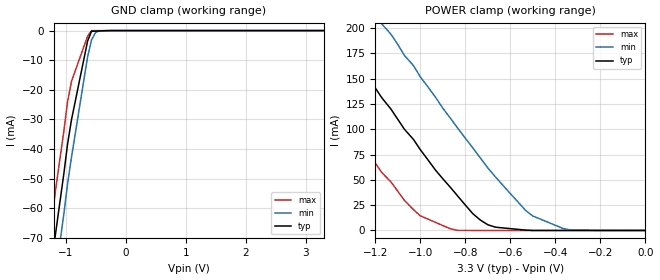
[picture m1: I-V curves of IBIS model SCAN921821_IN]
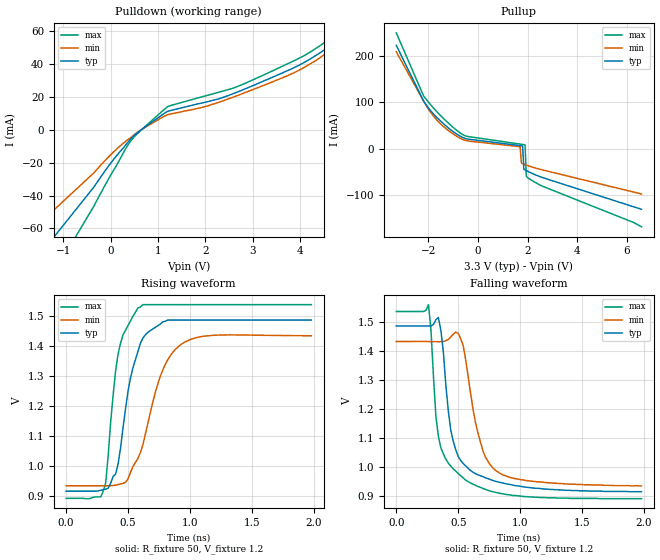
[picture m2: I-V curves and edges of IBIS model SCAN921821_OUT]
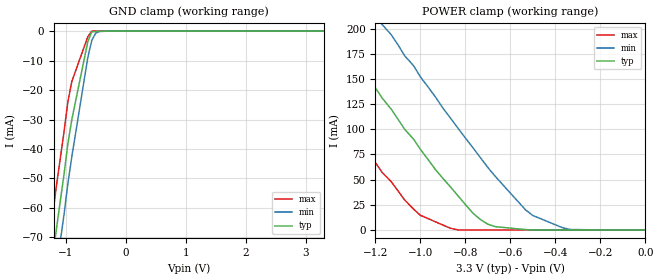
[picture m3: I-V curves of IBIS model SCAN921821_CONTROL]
|   National Semiconductor Corporation
|   IBIS Model of SCAN921821TSM
|   Dual 18-Bit BUS LVDS Serializer with Pre-emphasis,
|   IEEE 1149.1 (JTAG), and At-Speed BIST - 15-66 MHz
|   100 Ball FBGA Package
[IBIS Ver]   3.2
[Comment Char]   |_char
[File name]   scan921821tsm.ibs
[File Rev]   1.0
[Date]   04/06/04
[Source]
SPICE to IBIS Translation
[Notes]
Rev1.0 - Initial draft;
-The model cover zero pre-emphasis case only;
Created by dglisic;
[Disclaimer]
(C) Copyright National Semiconductor Corporation 2002
   All rights reserved
   National Semiconductor Corporation hereby grants
the user of this IBIS model a non-exclusive, nontransferable
license to use this IBIS model under the following terms.
Before using this IBIS model, the user should read this
license.  If the user does not accept these terms,  the
IBIS model should be returned to National within 30 days.
   The user is granted this license only to use the
IBIS model and is not granted rights to sell, load, rent,
lease or license the IBIS model in whole or in part, or in
modified form to anyone other than user. User may modify
the IBIS model to suit its specific applications but rights
to derivative works and such modifications shall belong to
National.
   This IBIS model is provided on an "AS IS" basis and
National makes absolutely no warranty with respect to the
information contained herein.NATIONAL DISCLAIMS AND CUSTOMER
WAIVES ALL WARRANTIES, EXPRESS OR IMPLIED, INCLUDING
WARRANTIES OF MERCHANTABILITY OR FITNESS FOR A PARTICULAR
PURPOSE. The entire risk as to quality and performance is
with the Customer. ACCORDINGLY, IN NO EVENT SHALL THE
COMPANY BE LIABLE FOR ANY DAMAGES, WHETHER IN CONTRACT OR
TORT,INCLUDING ANY LOST PROFITS OR OTHER INCIDENTAL,
CONSEQUENTIAL, EXEMPLARY, OR PUNITIVE DAMAGES ARISING OUT
OF THE USE OR APPLICATION OF THE IBIS model provided in
this package.Further, National reserves the right to make
changes without notice to any product herein to improve
reliability, function, or design. National does not convey
any license under patent rights or any other intellectual
property rights, including those of third parties.
   National is not obligated to provide maintenance or support
for the licensed IBIS model.
Contact National at ATTN:INTERFACE APPLICATIONS/IBIS MODELS.
5 Foden Road, M/S 03-03, South Porltand, ME 04106
(207) 541-6031
[Copyright]
(c) Copyright 2002 National Semiconductor Corp.
[Component]   SCAN921821TSM
Si_location Pin
Timing_location Pin
[Manufacturer]   National Semiconductor Corp.
[Package]
|   TYP   MIN   MAX
R_pkg   0.451   0.428   0.605
L_pkg   3.235nH   2.783n   4.687n
C_pkg   0.090pF   0.075p   0.158p
[Pin]   signal_name   model_name   R_pin   L_pin   C_pin
A1   BISTB   SCAN921821_CONTROL   0.451   3.235n  0.090p
A2   PVSS   GND   0.451   3.235n  0.090p
A3   DOUTBN  SCAN921821_OUT   0.494   3.212n  0.082p
A4   AVDD   POWER   0.469   3.235n  0.090p
A5   ENB   SCAN921821_CONTROL   0.431   2.989n  0.087p
A6   AVDD   POWER   0.429   3.125n  0.087p
A7   DOUTAN  SCAN921821_OUT   0.429   3.199n  0.087p
A8   DOUTAP  SCAN921821_OUT   0.445   3.581n  0.089p
A9   AVDD   POWER   0.463   3.856n  0.108p
A10   ENA   SCAN921821_CONTROL   0.451   3.235n  0.090p
B1   DINB16  SCAN921821_IN   0.451   3.235n  0.090p
B2   SYNCB   SCAN921821_CONTROL   0.451   3.235n  0.090p
B3   AVDD   POWER   0.588   3.928n  0.158p
B4   DOUTBP  SCAN921821_OUT   0.485   2.948n  0.082p
B5   AVDD   POWER   0.456   3.235n  0.090p
B6   PEMB1   SCAN921821_CONTROL   0.454   3.235n  0.090p
B7   AVSS   GND   0.428   3.235n  0.090p
B8   PEMB0   SCAN921821_CONTROL   0.477   3.235n  0.090p
B9   PEMA1   SCAN921821_CONTROL   0.451   3.235n  0.090p
B10   BISTA   SCAN921821_CONTROL   0.451   3.235n  0.090p
C1   DINB14  SCAN921821_IN   0.451   3.235n  0.090p
C2   DVDD   POWER   0.451   3.235n  0.090p
C3   DVSS   GND   0.451   3.235n  0.090p
C4   AVSS   GND   0.605   3.235n  0.090p
C5   AVSS   GND   0.544   3.235n  0.090p
C6   AVSS   GND   0.464   3.235n  0.090p
C7   AVDD   POWER   0.447   3.235n  0.090p
C8   PEMA2   SCAN921821_CONTROL   0.451   3.235n  0.090p
C9   SYNCA   SCAN921821_CONTROL   0.451   3.235n  0.090p
C10   DINA16  SCAN921821_IN   0.451   3.235n  0.090p
D1   DINB13  SCAN921821_IN   0.556   3.235n  0.090p
D2   DINB12  SCAN921821_IN   0.451   3.235n  0.090p
D3   DINB17  SCAN921821_IN   0.451   3.235n  0.090p
D4   DVDD   POWER   0.451   3.235n  0.090p
D5   PVDD   POWER   0.451   3.235n  0.090p
D6   PEMA0   SCAN921821_CONTROL   0.451   3.235n  0.090p
D7   AVSS   GND   0.451   3.235n  0.090p
D8   DINA17  SCAN921821_IN   0.451   3.235n  0.090p
D9   DINA15  SCAN921821_IN   0.451   3.235n  0.090p
D10   DINA13  SCAN921821_IN   0.451   3.235n  0.090p
E1   DINB11  SCAN921821_IN   0.451   3.235n  0.090p
E2   DINB9   SCAN921821_IN   0.451   3.235n  0.090p
E3   DINB15  SCAN921821_IN   0.451   3.235n  0.090p
E4   DVSS   GND   0.451   3.235n  0.090p
E5   DINB8   SCAN921821_IN   0.451   3.235n  0.090p
E6   PEMB2   SCAN921821_CONTROL   0.600   3.235n  0.090p
E7   DVSS   GND   0.451   3.235n  0.090p
E8   DINA14  SCAN921821_IN   0.451   3.235n  0.090p
E9   DINA12  SCAN921821_IN   0.451   3.235n  0.090p
E10   DINA9   SCAN921821_IN   0.451   3.235n  0.090p
F1   DINB10  SCAN921821_IN   0.451   3.235n  0.090p
F2   DINB7   SCAN921821_IN   0.451   3.235n  0.090p
F3   DINB5   SCAN921821_IN   0.451   3.235n  0.090p
F4   DVSS   GND   0.451   3.235n  0.090p
F5   PVDD   POWER   0.451   3.235n  0.090p
F6   DINA11  SCAN921821_IN   0.451   3.235n  0.090p
F7   DVSS   GND   0.451   3.235n  0.090p
F8   DINA4   SCAN921821_IN   0.451   3.235n  0.090p
F9   DINA10  SCAN921821_IN   0.451   3.235n  0.090p
F10   DINA8   SCAN921821_IN   0.451   3.235n  0.090p
G1   DINB6   SCAN921821_IN   0.451   3.235n  0.090p
G2   DINB4   SCAN921821_IN   0.451   3.235n  0.090p
G3   DINB2   SCAN921821_IN   0.451   3.235n  0.090p
G4   DVSS   GND   0.451   3.235n  0.090p
G5   DVDD   POWER   0.451   3.235n  0.090p
G6   DVDD   POWER   0.451   3.235n  0.090p
G7   DINA1   SCAN921821_IN   0.451   3.235n  0.090p
G8   DINA2   SCAN921821_IN   0.451   3.235n  0.090p
G9   DINA7   SCAN921821_IN   0.451   3.235n  0.090p
G10   DINA6   SCAN921821_IN   0.451   3.235n  0.090p
H1   DINB3   SCAN921821_IN   0.451   3.235n  0.090p
H2   DINB1   SCAN921821_IN   0.451   3.235n  0.090p
H3   TxCLK   SCAN921821_IN   0.451   3.235n  0.090p
H4   DVSS   GND   0.451   3.235n  0.090p
H5   TCK   SCAN921821_CONTROL   0.451   3.235n  0.090p
H6   PVDD   POWER   0.451   3.235n  0.090p
H7   PVSS   GND   0.451   3.235n  0.090p
H8   DVSS   GND   0.451   3.235n  0.090p
H9   DINA0   SCAN921821_IN   0.451   3.235n  0.090p
H10   DINA5   SCAN921821_IN   0.451   3.235n  0.090p
J1   DINB0   SCAN921821_IN   0.451   3.235n  0.090p
J2   PWDNA*  SCAN921821_CONTROL   0.451   3.235n  0.090p
J3   DVDD   POWER   0.451   3.235n  0.090p
J4   TRST*   SCAN921821_CONTROL   0.451   3.235n  0.090p
J5   PVDD   POWER   0.451   3.235n  0.090p
J6   PVSS   GND   0.451   3.235n  0.090p
J7   PVDD   POWER   0.451   3.235n  0.090p
J8   NC   NC   0.451   3.235n  0.090p
J9   DVDD   POWER   0.451   3.235n  0.090p
J10   DINA3   SCAN921821_IN   0.451   3.235n  0.090p
K1   DVSS   GND   0.451   3.235n  0.090p
K2   TDI   SCAN921821_CONTROL   0.451   3.235n  0.090p
K3   TMS   SCAN921821_CONTROL   0.451   3.235n  0.090p
K4   DVSS   GND   0.451   3.235n  0.090p
K5   TDO   NC   0.451   3.235n  0.090p
K6   DVDD   POWER   0.451   3.235n  0.090p
K7   PVSS   GND   0.451   3.235n  0.090p
K8   PVSS   GND   0.451   3.235n  0.090p
K9   PWDNB*  SCAN921821_CONTROL   0.451   3.235n  0.090p
K10   DVDD   POWER   0.451   3.235n  0.090p
[Diff Pin] inv_pin   vdiff   tdelay_typ   tdelay_min   tdelay_max
| The '+' pin is Diff_pin and the '-' pin is the inv_pin
| Receiver Vth = +/-100mV
A8   A7   NA   0   0   0
B4   A3   NA   0   0   0
| Models and submodels in the file (3): SCAN921821_IN (Input), SCAN921821_OUT (Output), SCAN921821_CONTROL (Input)
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[Model]   SCAN921821_IN
Model_type Input
Vinh=2.0
Vinl=0.8
C_comp   4.0pF   4.0pF   4.0pF
[Temperature Range] 25   85   -40
[Voltage Range]   3.3   3.15   3.45
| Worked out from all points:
|   GND clamp passes 1 mA (typ) near -0.58 V on its own axis
|   POWER clamp passes 1 mA (typ) near -0.56 V on its own axis
[GND Clamp]
|V(groundclamp)   I(typ)   I(min)   I(max)
-3.3V     -416mA     -429mA     -402mA
-1.3V     -89.7mA    -104mA     -74.9mA
-1.23V    -79.3mA    -93mA      -64.5mA
-1.17V    -69.1mA    -82.7mA    -54.4mA
-1.1V     -58.8mA    -72.5mA    -44.3mA
-1.03V    -48.6mA    -62.2mA    -34.2mA
-967mV    -38.4mA    -51.9mA    -24.1mA
-900mV    -30mA      -42.6mA    -17.1mA
-633mV    -3.57mA    -8.92mA    -1.9mA
-567mV    -239uA     -3.14mA    -420nA
-433mV    -133uA     -61.9uA    -233nA
3.3V      21.4pA     6.6nA      19.4pA
[POWER Clamp]
|Vtable   I(typ)   I(min)   I(max)
-3.3V     826mA      900mA      750mA
-1.63V    280mA      354mA      203mA
-1.6V     269mA      344mA      193mA
-1.37V    194mA      268mA      118mA
-1.17V    131mA      204mA      57.1mA
-1.13V    120mA      194mA      48mA
-1V       80mA       152mA      14.5mA
-833mV    33.9mA     101mA      60uA
-700mV    5.68mA     61.9mA     6.68uA
-533mV    372uA      20mA       1.71nA
-366mV    1.1uA      2.03mA     12.8pA
0V        6.66pA     6.59nA     6.3pA
[Model]   SCAN921821_OUT
Model_type Output
Vref=1.2
Vmeas=1.2
Rref=50   | 100 Ohms Across Outputs OUTP and OUTM
Cref=0p
C_comp   3.122pF   3.122pF   3.122pF
[Temperature Range] 25   85   -40
[Voltage Range]   3.3   3.15   3.45
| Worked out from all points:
|   slope of the pulldown table from 0 to 0.495 V, typ, clamps not added: 29.3 ohm
|   slope of the pullup table from 0 to 0.495 V, typ, clamps not added: 151 ohm
|   falling waveform, R_fixture 50, V_fixture 1.2: 20-80 % time 126ps typ, 147ps min, 123ps max; typ from 1.49 V to 0.916 V
|   rising waveform, R_fixture 50, V_fixture 1.2: 20-80 % time 144ps typ, 207ps min, 102ps max; typ from 0.917 V to 1.49 V
[Pullup]
|Vtable   I(typ)   I(min)   I(max)
-3.3V     223mA      209mA      250mA
-2.2V     103mA      103mA      114mA
-1.6V     64.1mA     58.2mA     76.1mA
-900mV    32.8mA     28mA       41.2mA
1.7V      6.41mA     4.1mA      9.71mA
1.75V     6.07mA     -31mA      9.32mA
1.8V      5.74mA     -32.6mA    8.93mA
1.85V     -44.3mA    -33.6mA    8.54mA
1.9V      -46.2mA    -34.6mA    8.15mA
1.95V     -47.6mA    -35.6mA    -59.6mA
2V        -48.9mA    -36.6mA    -62.7mA
6.6V      -131mA     -98mA      -169mA
[Pulldown]
|V(pulldown)   I(typ)   I(min)   I(max)
-3.3V     -141mA     -105mA     -188.8mA
-358mV    -35mA      -26.3mA    -46.65mA
423mV     -5.55mA    -4.77mA    -6.829mA
1.204V    11.3mA     9.21mA     14.14mA
2.056V    17.2mA     14.6mA     21.07mA
2.624V    22.4mA     20.3mA     25.75mA
3.902V    38.2mA     35.1mA     42.43mA
4.541V    49.1mA     46.5mA     53.61mA
4.683V    52.1mA     51.3mA     56.65mA
4.896V    57.4mA     63.7mA     61.48mA
5.038V    62.9mA     74.8mA     65.14mA
6.6V      227mA      228mA      232.6mA
[Falling Waveform]
R_fixture=50
V_fixture=1.2
V_fixture_min=1.2
V_fixture_max=1.2
0s        1.487V     1.434V     1.537V
260ps     1.487V     1.434V     1.561V
320ps     1.509V     1.433V     1.175V
340ps     1.517V     1.433V     1.107V
440ps     1.129V     1.45V      1.004V
500ps     1.037V     1.462V     979mV
560ps     1.005V     1.372V     956mV
660ps     974mV      1.118V     934mV
800ps     952mV      990mV      914mV
1.98ns    916mV      936mV      892mV
[Rising Waveform]
R_fixture=50
V_fixture=1.2
V_fixture_min=1.2
V_fixture_max=1.2
0s        917mV      935mV      893mV
300ps     922mV      935mV      917mV
320ps     924mV      935mV      945mV
380ps     966mV      936mV      1.237V
420ps     1.008V     939mV      1.374V
500ps     1.25V      958mV      1.468V
580ps     1.382V     1.026V     1.527V
760ps     1.473V     1.299V     1.538V
920ps     1.487V     1.403V     1.538V
1.98ns    1.487V     1.435V     1.538V
[Ramp]
|   typ   min   max
dV/dt_r   320mV/.213ns   310mV/.222ns   330mV/.150ns
dV/dt_f   320mv/.192ns   310mv/.241ns   330mv/.156ns
R_load=50
|[End   SCAN921821_OUT
[Model]   SCAN921821_CONTROL
Model_type Input
Vinh=2.0
Vinl=0.8
C_comp   4.0pF   4.0pF   4.0pF
[Temperature Range] 25   85   -40
[Voltage Range]   3.3   3.15   3.45
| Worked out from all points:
|   GND clamp passes 1 mA (typ) near -0.58 V on its own axis
|   POWER clamp passes 1 mA (typ) near -0.56 V on its own axis
[GND Clamp]
-3.3V     -416mA     -429mA     -402mA
-1.3V     -89.7mA    -104mA     -74.9mA
-1.23V    -79.3mA    -93mA      -64.5mA
-1.17V    -69.1mA    -82.7mA    -54.4mA
-1.1V     -58.8mA    -72.5mA    -44.3mA
-1.03V    -48.6mA    -62.2mA    -34.2mA
-967mV    -38.4mA    -51.9mA    -24.1mA
-900mV    -30mA      -42.6mA    -17.1mA
-633mV    -3.57mA    -8.92mA    -1.9mA
-567mV    -239uA     -3.14mA    -420nA
-433mV    -133uA     -61.9uA    -233nA
3.3V      21.4pA     6.6nA      19.7pA
[POWER Clamp]
-3.3V     826mA      900mA      750mA
-1.63V    280mA      354mA      203mA
-1.6V     269mA      344mA      193mA
-1.37V    194mA      268mA      118mA
-1.17V    131mA      204mA      57.1mA
-1.13V    120mA      194mA      48mA
-1V       80mA       152mA      14.5mA
-833mV    33.9mA     101mA      60uA
-700mV    5.68mA     61.9mA     6.68uA
-533mV    372uA      20mA       1.71nA
-366mV    1.1uA      2.03mA     12.8pA
0V        6.66pA     6.59nA     6.3pA
